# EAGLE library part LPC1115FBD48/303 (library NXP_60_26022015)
32-bit ARM Cortex-M0 microcontroller; up to 64 kB flash and 8 kB SRAM The LPC1110/11/12/13/14/15 are a ARM Cortex-M0 based, low-cost 32-bit MCU family, designed for 8/16-bit microcontroller applications, offering performance, low power, simple instruction set and memory addressing together with reduced code size compared to existing 8/16-bit architectures. The LPC1110/11/12/13/14/15 operate at CPU frequencies of up to 50 MHz. The peripheral complement of the LPC1110/11/12/13/14/15 includes up to 64 kB of flash memory, up to 8 kB of data memory, one Fast-mode Plus I 2 C-bus interface, one RS-485/EIA-485 UART, up to two SPI interfaces with SSP features, four general purpose counter/timers, a 10-bit ADC, and up to 42 general purpose I/O pins. Remark: The LPC111x series consists of the LPC1100 series (parts LPC111x/101/201/301), LPC1100L series (parts LPC111x/002/102/202/302), and the LPC1100XL series (parts LPC111x/103/203/303/323/333). The LPC1100L and LPC1100XL series include the power profiles, a windowed watchdog timer, and a configurable open-drain mode. AAL Eindhoven MK
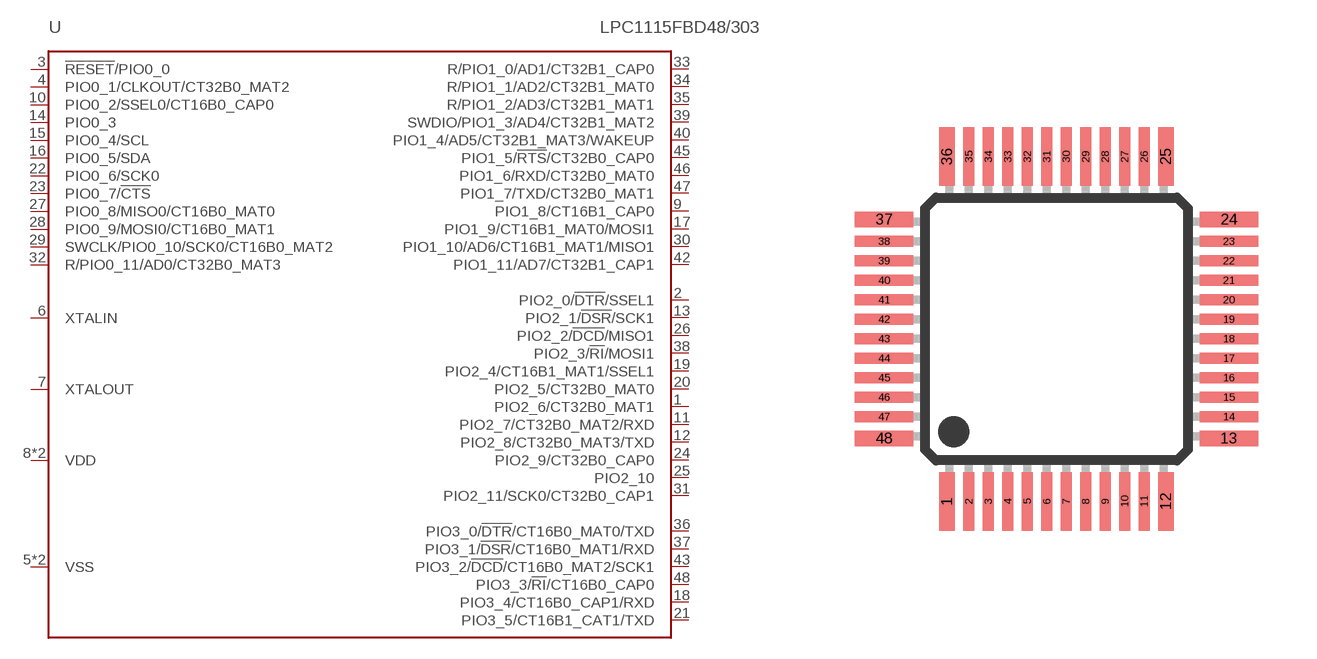
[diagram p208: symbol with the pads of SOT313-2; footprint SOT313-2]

Designator prefix U

## LPC1115FBD48/303 (ADC: 8; FLASH: 64kB; GPIO: 42; PWR_PROFILES: yes; SERIES: LPC1100XL; SPI: 2; SRAM: 8kB)  [SOT313-2]
1  PIO2_6/CT32B0_MAT1
2  PIO2_0/!DTR!/SSEL1
3  !RESET!/PIO0_0
4  PIO0_1/CLKOUT/CT32B0_MAT2
5  VSS  pwr
6  XTALIN  in
7  XTALOUT  out
8  VDD  pwr
9  PIO1_8/CT16B1_CAP0
10  PIO0_2/SSEL0/CT16B0_CAP0
11  PIO2_7/CT32B0_MAT2/RXD
12  PIO2_8/CT32B0_MAT3/TXD
13  PIO2_1/!DSR!/SCK1
14  PIO0_3
15  PIO0_4/SCL
16  PIO0_5/SDA
17  PIO1_9/CT16B1_MAT0/MOSI1
18  PIO3_4/CT16B0_CAP1/RXD
19  PIO2_4/CT16B1_MAT1/SSEL1
20  PIO2_5/CT32B0_MAT0
21  PIO3_5/CT16B1_CAT1/TXD
22  PIO0_6/SCK0
23  PIO0_7/!CTS!
24  PIO2_9/CT32B0_CAP0
25  PIO2_10
26  PIO2_2/!DCD!/MISO1
27  PIO0_8/MISO0/CT16B0_MAT0
28  PIO0_9/MOSI0/CT16B0_MAT1
29  SWCLK/PIO0_10/SCK0/CT16B0_MAT2
30  PIO1_10/AD6/CT16B1_MAT1/MISO1
31  PIO2_11/SCK0/CT32B0_CAP1
32  R/PIO0_11/AD0/CT32B0_MAT3
33  R/PIO1_0/AD1/CT32B1_CAP0
34  R/PIO1_1/AD2/CT32B1_MAT0
35  R/PIO1_2/AD3/CT32B1_MAT1
36  PIO3_0/!DTR!/CT16B0_MAT0/TXD
37  PIO3_1/!DSR!/CT16B0_MAT1/RXD
38  PIO2_3/!RI!/MOSI1
39  SWDIO/PIO1_3/AD4/CT32B1_MAT2
40  PIO1_4/AD5/CT32B1_MAT3/WAKEUP
41  VSS  pwr
42  PIO1_11/AD7/CT32B1_CAP1
43  PIO3_2/!DCD!/CT16B0_MAT2/SCK1
44  VDD  pwr
45  PIO1_5/!RTS!/CT32B0_CAP0
46  PIO1_6/RXD/CT32B0_MAT0
47  PIO1_7/TXD/CT32B0_MAT1
48  PIO3_3/!RI!/CT16B0_CAP0

## Footprint SOT313-2 (pad centres in mm)
SOT313-2 LQFP48: plastic low profile quad flat package; 48 leads; body 7 x 7 x 1.4 mm JEDEC: MS-026 IEC: 136E05 Footprint according to NXP SOT313-2 specification, however the cornerpins are 0.4mm in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
smd 0.4 x 1.5: 1 -2.81,-4.425; 12 2.81,-4.425; 25 2.81,4.425; 36 -2.81,4.425
smd 0.28 x 1.5: 2 -2.25,-4.425; 3 -1.75,-4.425; 4 -1.25,-4.425; 5 -0.75,-4.425; 6 -0.25,-4.425; 7 0.25,-4.425; 8 0.75,-4.425; 9 1.25,-4.425; 10 1.75,-4.425; 11 2.25,-4.425; 26 2.25,4.425; 27 1.75,4.425; 28 1.25,4.425; 29 0.75,4.425; 30 0.25,4.425; 31 -0.25,4.425; 32 -0.75,4.425; 33 -1.25,4.425; 34 -1.75,4.425; 35 -2.25,4.425
smd 1.5 x 0.4: 13 4.425,-2.81; 24 4.425,2.81; 37 -4.425,2.81; 48 -4.425,-2.81
smd 1.5 x 0.28: 14 4.425,-2.25; 15 4.425,-1.75; 16 4.425,-1.25; 17 4.425,-0.75; 18 4.425,-0.25; 19 4.425,0.25; 20 4.425,0.75; 21 4.425,1.25; 22 4.425,1.75; 23 4.425,2.25; 38 -4.425,2.25; 39 -4.425,1.75; 40 -4.425,1.25; 41 -4.425,0.75; 42 -4.425,0.25; 43 -4.425,-0.25; 44 -4.425,-0.75; 45 -4.425,-1.25; 46 -4.425,-1.75; 47 -4.425,-2.25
